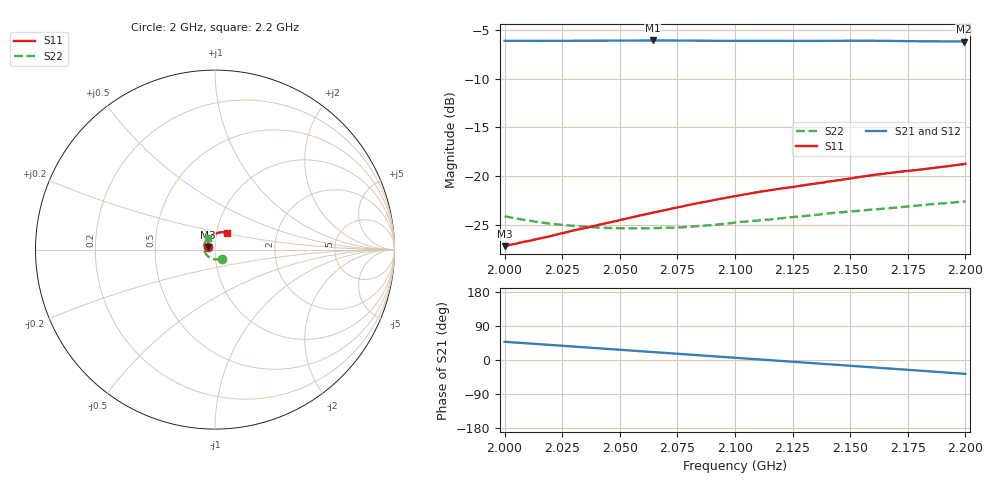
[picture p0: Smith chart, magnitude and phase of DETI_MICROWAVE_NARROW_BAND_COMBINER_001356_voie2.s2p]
! 12/28/2020 4:22:01 PM
! \\DETI-AD\SERVEUR COMMUN\0\01 - PRODUIT\0 01 356 - COMBINEUR 4 VOIES BANDE S 800 WATTS\81 -PROCES VERBAL DE CONTROLE\MESURES\07 - S2P\VOIE2.S2P
! CHANNEL.1
! TR.MEASUREMENT
! CORRECTED.DATA
# GHZ S RI R 50.0
! FREQ.GHZ  S11RE  S11IM  S21RE  S21IM  S12RE  S12IM  S22RE  S22IM
!; PortSelection: Port_12
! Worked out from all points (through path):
!   1000 points, 2 GHz to 2.2 GHz, reference 50 ohm
!   highest |S21| = -6.05 dB at 2.064 GHz (marker M1); lowest = -6.2 dB at 2.199 GHz (marker M2)
!   lowest |S11| = -27.2 dB at 2 GHz (marker M3), VSWR 1.09, Z = 46 + j1.38 ohm
!   |S11| at or under -10 dB: start of sweep to end of sweep
!   |S22| runs from -25.4 to -22.6 dB; largest |S21 - S12| = 0.0025
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2  -0.0409 0.0149  0.3317 0.3694  0.3315 0.3698  0.0369 -0.05
2.006807  -0.0409 0.0198  0.3497 0.3522  0.3496 0.3524  0.0294 -0.0523
2.016016  -0.04 0.0264  0.3722 0.328  0.3724 0.3281  0.019 -0.0543
2.024825  -0.039 0.0323  0.3927 0.3036  0.393 0.3034  0.0092 -0.0553
2.033433  -0.0375 0.0383  0.4115 0.2785  0.4117 0.2783  -0.00014 -0.055
2.044845  -0.0346 0.0458  0.4338 0.2435  0.4339 0.2427  -0.012 -0.0527
2.058458  -0.0306 0.0546  0.4568 0.1985  0.4564 0.1979  -0.025 -0.0475
2.064264  -0.0285 0.0582  0.4654 0.1786  0.4643 0.1783  -0.0303 -0.0445
2.066667  -0.0276 0.0596  0.4684 0.1703  0.4675 0.1697  -0.0323 -0.0433
2.077277  -0.0232 0.0658  0.4799 0.1326  0.4789 0.1325  -0.0404 -0.0366
2.091892  -0.0162 0.0739  0.4901 0.0796  0.4896 0.0797  -0.0499 -0.0258
2.1001  -0.0116 0.0779  0.4936 0.0496  0.4933 0.0501  -0.0543 -0.0192
2.10991  -0.00588 0.0824  0.4959 0.0146  0.4959 0.0146  -0.058 -0.0108
2.115916  -0.00213 0.0847  0.4959 -0.00649  0.4957 -0.00685  -0.0596 -0.00557
2.133534  0.0098 0.0903  0.4908 -0.0702  0.4897 -0.0713  -0.0619 0.0106
2.140541  0.0151 0.0923  0.4866 -0.0962  0.4852 -0.097  -0.0618 0.017
2.150951  0.0234 0.0947  0.4785 -0.1341  0.4767 -0.1343  -0.0602 0.0265
2.16016  0.0307 0.0966  0.4681 -0.1663  0.4659 -0.1659  -0.0577 0.0346
2.166767  0.0362 0.097  0.4584 -0.1889  0.4565 -0.1878  -0.0551 0.0403
2.186987  0.0541 0.0961  0.4217 -0.2554  0.4215 -0.254  -0.0451 0.0561
2.199399  0.0656 0.0947  0.3968 -0.2914  0.3966 -0.2906  -0.0369 0.0641
2.2  0.0661 0.0947  0.3956 -0.2933  0.3954 -0.2924  -0.0364 0.0644
